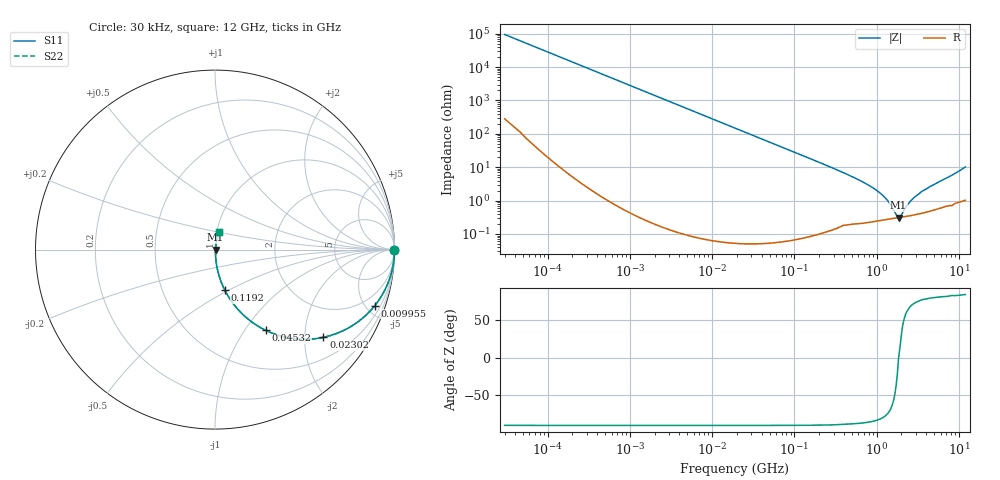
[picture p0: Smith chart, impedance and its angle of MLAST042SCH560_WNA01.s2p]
! MLAST042SCH560_WNA01  S-PARAMETER MODEL  ( General Type )
! Model Generated by TAIYO YUDEN Corporation (http://www.ty-top.com)
! Version 1.0
! TAIYO YUDEN Control No. 150820
! Copyright(c) 2015 TAIYO YUDEN CO.,LTD. All Rights Reserved.
! Product Description (link to TY-COMPAS)
! https://ds.yuden.co.jp/TYCOMPAS/or/detail?pn=MLAST042SCH560JWNA01&u=M
! Products Name : Multilayer Ceramic Capacitors
! Characteristics :
!  Capacitance : 56 pF , Rated Voltage : 25V , TCC : CH / C0H
!  Case Size : 0.4 x 0.2 / 0.016 x 0.008 [mm/inch] , Thickness : 0.2 / 0.008 [mm/inch]
!  (Conditions: Temperature = 25 degC , DC Bias Current/Voltage = 0A / 0V)
! External Node Assignments :
!  1  o---| |---o  2
! GND o---------o GND
! Frequency Range : 0.03MHz  -  12000MHz  [ 401 STEP ]
# MHz S RI R 50
! Freq[MHz].  S11 Real  S11 Imag  S21 Real  S21 Imag  S12 Real  S12 Imag  S22 Real  S22 Imag
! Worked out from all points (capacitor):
!   401 points, 30 kHz to 12 GHz, reference 50 ohm
!   read as one part in series: C = 56 pF near 32 kHz
!   lowest |Z| = 309 mohm at 1.849 GHz (marker M1)
!   series resonance near 1.85 GHz, so ESL is about 130 pH
!   S11 on the Smith chart (normalised r, x): 30 kHz: open; 9.955 MHz: 1.00, -5.71; 23.02 MHz: 1.00, -2.47; 45.32 MHz: 1.00, -1.25; 119.2 MHz: 1.00, -0.47; 12 GHz: 1.02, +0.20
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0.03  1 -0.00106  4.25e-06 0.00106  4.25e-06 0.00106  1 -0.00106
0.260295  0.9999 -0.00916  8.66e-05 0.00916  8.66e-05 0.00916  0.9999 -0.00916
2.258455  0.9937 -0.079  0.00629 0.079  0.00629 0.079  0.9937 -0.079
4.897055  0.9711 -0.1673  0.0289 0.1673  0.0289 0.1673  0.9711 -0.1673
9.95516  0.8907 -0.312  0.1093 0.312  0.1093 0.312  0.8907 -0.312
18.97367  0.6916 -0.4617  0.3084 0.4617  0.3084 0.4617  0.6916 -0.4617
23.02407  0.6036 -0.4889  0.3964 0.4889  0.3964 0.4889  0.6036 -0.4889
45.32004  0.2822 -0.4496  0.7178 0.4496  0.7178 0.4496  0.2822 -0.4496
71.18072  0.1375 -0.3437  0.8625 0.3437  0.8625 0.3437  0.1375 -0.3437
119.2463  0.0539 -0.2244  0.9461 0.2244  0.9461 0.2244  0.0539 -0.2244
164.6252  0.0293 -0.1661  0.9707 0.1661  0.9707 0.1661  0.0293 -0.1661
419.4166  0.00595 -0.0638  0.9941 0.0638  0.9941 0.0638  0.00595 -0.0638
749.4426  0.00317 -0.0316  0.9968 0.0316  0.9968 0.0316  0.00317 -0.0316
1103.571  0.00279 -0.0166  0.9972 0.0166  0.9972 0.0166  0.00279 -0.0166
1428.372  0.00285 -0.00809  0.9972 0.00809  0.9972 0.00809  0.00285 -0.00809
1733.294  0.00301 -0.00211  0.997 0.00211  0.997 0.00211  0.00301 -0.00211
1848.769  0.00308 -9.95e-06  0.9969 9.95e-06  0.9969 9.95e-06  0.00308 -9.95e-06
1971.936  0.00317 0.00146  0.9968 -0.00146  0.9968 -0.00146  0.00317 0.00146
2316.96  0.00341 0.00609  0.9966 -0.00609  0.9966 -0.00609  0.00341 0.00609
2635.962  0.00366 0.00954  0.9963 -0.00954  0.9963 -0.00954  0.00366 0.00954
3411.775  0.00437 0.017  0.9956 -0.017  0.9956 -0.017  0.00437 0.017
12000  0.02 0.0981  0.98 -0.0981  0.98 -0.0981  0.02 0.0981
